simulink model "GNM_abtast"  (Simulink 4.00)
settings: Solver=ode45  StartTime=0.0  StopTime=0.2  RelTol=1e-3
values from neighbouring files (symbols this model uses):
  CE = (2*NA/pi)*2*pi    (= 240)    [GNM_abtast_ini.m]
  CM = 2*NA/pi    (= 38.1971863421)    [GNM_abtast_ini.m]
  Fpwm = 5000    [GNM_abtast_ini.m]
  Imax = 20    [GNM_abtast_ini.m]
  J = 0.012    [GNM_abtast_ini.m]
  LA = 0.004    [GNM_abtast_ini.m]
  Mw = 10    [GNM_abtast_ini.m]
  N_soll = 1000 / 60    (= 16.6666666667)    [GNM_abtast_ini.m]
  psi = 0.04    [GNM_abtast_ini.m]
  RA = 0.25    [GNM_abtast_ini.m]
  TnAd = 8*Tsn/2    (= 0.0032)    [GNM_abtast_ini.m]
  Tsi = 0.0008    [GNM_abtast_ini.m]
  Tsn = 0.0008    [GNM_abtast_ini.m]
  TstrA = 1 / Fpwm / 2    (= 0.0001)    [GNM_abtast_ini.m]
  Umax = 200    [GNM_abtast_ini.m]
  VnAd = 2*pi*J/(4*Tsn/2*CM*psi)    (= 30.8425137534)    [GNM_abtast_ini.m]
undefined symbols (not defined in the file or in its folder): Ad, Bd
libraries: simulink3 x1

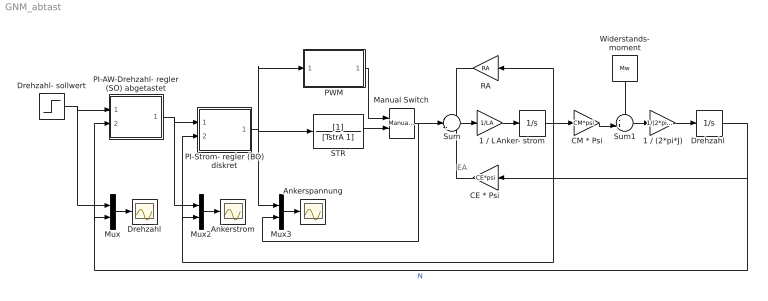
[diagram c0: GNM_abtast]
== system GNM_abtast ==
  note: EA
  " Widerstands-  moment" : Constant  Orientation=down  Value=Mw
  1 / (2*pi*J) : Gain  Gain=1/(2*pi*J)  Multiplication=Element-wise(K.*u)  SaturateOnIntegerOverflow=on
  1 / LA : Gain  Gain=1/LA  Multiplication=Element-wise(K.*u)  SaturateOnIntegerOverflow=on
  Anker- strom : Integrator  ExternalReset=none  InitialConditionSource=internal  InitialCondition=0  LimitOutput=off  UpperSaturationLimit=inf  LowerSaturationLimit=-inf  ShowSaturationPort=off  ShowStatePort=off  AbsoluteTolerance=auto
  Ankerspannung : Scope
  Ankerstrom : Scope
  "CE * Psi " : Gain  Orientation=left  Gain=CE*psi  Multiplication=Element-wise(K.*u)  SaturateOnIntegerOverflow=on
  CM * Psi : Gain  Gain=CM*psi  Multiplication=Element-wise(K.*u)  SaturateOnIntegerOverflow=on
  Drehzahl : Scope
  "Drehzahl " : Integrator  ExternalReset=none  InitialConditionSource=internal  InitialCondition=0  LimitOutput=off  UpperSaturationLimit=inf  LowerSaturationLimit=-inf  ShowSaturationPort=off  ShowStatePort=off  AbsoluteTolerance=auto
  Drehzahl- sollwert : Step  Time=0.05  Before=0  After=N_soll  SampleTime=0
  Manual Switch : simulink3/Nonlinear/Manual Switch  sw=0  action=0
  Mux : Mux  Inputs=2
  Mux2 : Mux  Inputs=2
  Mux3 : Mux  Inputs=2
  PI-AW-Drehzahl- regler (SO) abgetastet : Subsystem
  PI-Strom- regler (BO) diskret : Subsystem
  PWM : Subsystem
  RA : Gain  Orientation=left  Gain=RA  Multiplication=Element-wise(K.*u)  SaturateOnIntegerOverflow=on
  STR : TransferFcn  Numerator=[1]  Denominator=[TstrA 1]  Realization=auto  AbsoluteTolerance=auto
  Sum : Sum  Inputs=-+-  SaturateOnIntegerOverflow=on
  Sum1 : Sum  Inputs=-+|  SaturateOnIntegerOverflow=on
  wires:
  RA/1 -> Sum/1
  Anker- strom/1 -> CM * Psi/1, RA/1, Mux2/2, PI-Strom- regler (BO) diskret/2(IA)
  Sum/1 -> 1 / LA/1
  1 / LA/1 -> Anker- strom/1
  CM * Psi/1 -> Sum1/2
  Sum1/1 -> 1 / (2*pi*J)/1
  1 / (2*pi*J)/1 -> "Drehzahl "/1
  " Widerstands-  moment"/1 -> Sum1/1
  "CE * Psi "/1 -> Sum/3
  PWM/1(UAist) -> Manual Switch/1
  STR/1 -> Manual Switch/2
  Mux/1 -> Drehzahl/1
  PI-AW-Drehzahl- regler (SO) abgetastet/1(IAsoll) -> PI-Strom- regler (BO) diskret/1(IAsoll), Mux2/1
  Mux2/1 -> Ankerstrom/1
  Mux3/1 -> Ankerspannung/1
  PI-Strom- regler (BO) diskret/1(UAsoll) -> Mux3/1, STR/1, PWM/1(UAsoll)
  Drehzahl- sollwert/1 -> Mux/1, PI-AW-Drehzahl- regler (SO) abgetastet/1(N_soll)
  Manual Switch/1 -> Sum/2, Mux3/2
  "Drehzahl "/1 -> "CE * Psi "/1, Mux/2, PI-AW-Drehzahl- regler (SO) abgetastet/2(N)  "N"

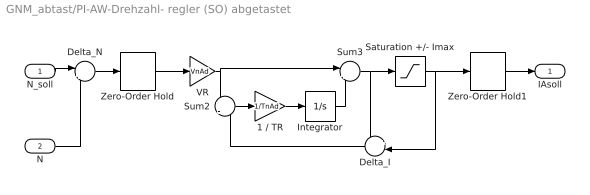
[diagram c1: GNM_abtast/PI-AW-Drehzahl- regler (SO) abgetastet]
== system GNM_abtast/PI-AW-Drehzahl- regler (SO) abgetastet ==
  N_soll : Inport  Port=1
  N : Inport  Port=2
  1 / TR : Gain  Gain=1/TnAd  Multiplication=Element-wise(K.*u)  SaturateOnIntegerOverflow=on
  Delta_I : Sum  Orientation=left  Inputs=+-|  SaturateOnIntegerOverflow=on
  Delta_N : Sum  Inputs=|+-  SaturateOnIntegerOverflow=on
  Integrator : Integrator  ExternalReset=none  InitialConditionSource=internal  InitialCondition=0  LimitOutput=off  UpperSaturationLimit=inf  LowerSaturationLimit=-inf  ShowSaturationPort=off  ShowStatePort=off  AbsoluteTolerance=auto
  Saturation +/- Imax : Saturate  UpperLimit=Imax  LowerLimit=-Imax  LinearizeAsGain=on
  Sum2 : Sum  Inputs=+|-  SaturateOnIntegerOverflow=on
  Sum3 : Sum  Inputs=|++  SaturateOnIntegerOverflow=on
  VR : Gain  Gain=VnAd  Multiplication=Element-wise(K.*u)  SaturateOnIntegerOverflow=on
  Zero-Order Hold : ZeroOrderHold  SampleTime=Tsn
  Zero-Order Hold1 : ZeroOrderHold  SampleTime=Tsn
  IAsoll : Outport  Port=1  InitialOutput=0
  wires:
  N_soll/1 -> Delta_N/1
  N/1 -> Delta_N/2
  Zero-Order Hold1/1 -> IAsoll/1
  Delta_N/1 -> Zero-Order Hold/1
  Integrator/1 -> Sum3/2
  Sum3/1 -> Saturation +/- Imax/1, Delta_I/1
  Sum2/1 -> 1 / TR/1
  VR/1 -> Sum2/1, Sum3/1
  Delta_I/1 -> Sum2/2
  1 / TR/1 -> Integrator/1
  Saturation +/- Imax/1 -> Delta_I/2, Zero-Order Hold1/1
  Zero-Order Hold/1 -> VR/1

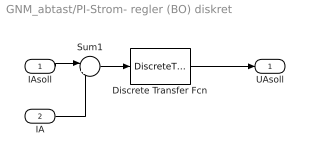
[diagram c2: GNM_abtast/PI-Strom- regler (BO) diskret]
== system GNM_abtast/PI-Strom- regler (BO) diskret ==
  IAsoll : Inport  Port=1
  IA : Inport  Port=2
  Discrete Transfer Fcn : DiscreteTransferFcn  Numerator=Bd  Denominator=Ad  SampleTime=Tsi  Realization=auto
  Sum1 : Sum  Inputs=|+-  SaturateOnIntegerOverflow=on
  UAsoll : Outport  Port=1  InitialOutput=0
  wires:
  IAsoll/1 -> Sum1/1
  IA/1 -> Sum1/2
  Sum1/1 -> Discrete Transfer Fcn/1
  Discrete Transfer Fcn/1 -> UAsoll/1

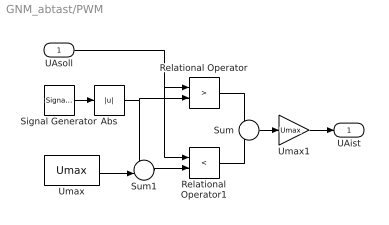
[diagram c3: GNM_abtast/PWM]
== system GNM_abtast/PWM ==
  UAsoll : Inport  Port=1
  Abs : Abs  SaturateOnIntegerOverflow=on
  Relational Operator : RelationalOperator  Operator=>
  Relational Operator1 : RelationalOperator  Operator=<
  Signal Generator : SignalGenerator  WaveForm=sawtooth  Amplitude=Umax  Frequency=Fpwm  Units=Hertz
  Sum : Sum  Inputs=+-  SaturateOnIntegerOverflow=on
  Sum1 : Sum  Inputs=+-|  SaturateOnIntegerOverflow=on
  Umax : Constant  Value=Umax
  Umax1 : Gain  Gain=Umax  Multiplication=Element-wise(K.*u)  SaturateOnIntegerOverflow=on
  UAist : Outport  Port=1  InitialOutput=0
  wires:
  Signal Generator/1 -> Abs/1
  Sum1/1 -> Relational Operator1/2
  UAsoll/1 -> Relational Operator1/1, Relational Operator/1
  Abs/1 -> Relational Operator/2, Sum1/1
  Umax/1 -> Sum1/2
  Relational Operator/1 -> Sum/1
  Relational Operator1/1 -> Sum/2
  Umax1/1 -> UAist/1
  Sum/1 -> Umax1/1
